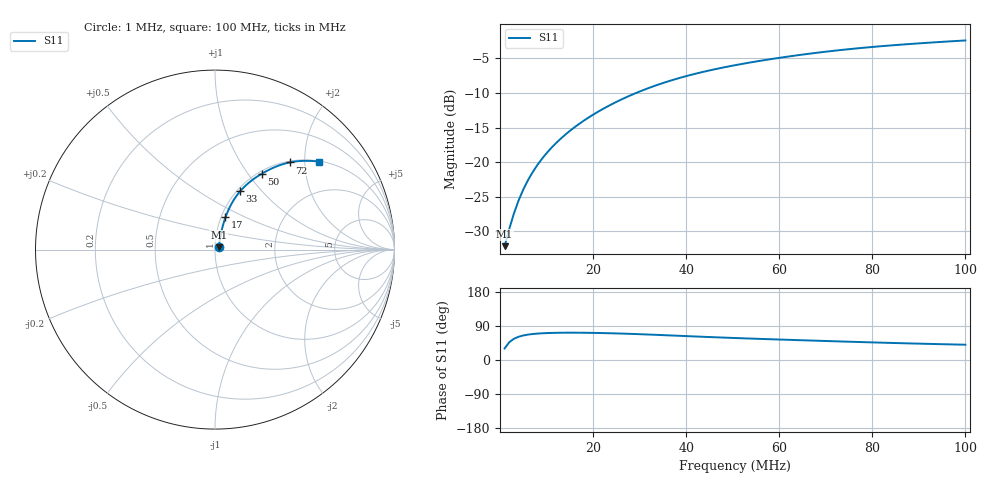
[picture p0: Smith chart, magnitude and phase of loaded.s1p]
# MHz S RI R 50.0
! SimSmith 18.4f
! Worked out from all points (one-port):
!   100 points, 1 MHz to 100 MHz, reference 50 ohm
!   lowest |S11| = -32.1 dB at 1 MHz (marker M1), VSWR 1.05, Z = 52.2 + j1.31 ohm
!   |S11| at or under -10 dB: start of sweep to 29.24 MHz
!   S11 on the Smith chart (normalised r, x): 1 MHz: 1.04, +0.03; 17 MHz: 1.05, +0.39; 33 MHz: 1.04, +0.77; 50 MHz: 1.04, +1.17; 72 MHz: 1.02, +1.69; 100 MHz: 1.02, +2.34
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1  0.0213 0.0125
2  0.0225 0.0241
3  0.0239 0.0353
4  0.0254 0.0464
5  0.027 0.0573
6  0.0289 0.068
7  0.0309 0.0786
8  0.033 0.0891
9  0.0353 0.0994
11  0.0403 0.1199
12  0.0429 0.13
14  0.0487 0.15
17  0.0585 0.1797
21  0.0739 0.2186
23  0.0828 0.2376
26  0.0978 0.2655
29  0.1148 0.2921
33  0.1401 0.3249
39  0.1822 0.3671
44  0.2188 0.3958
50  0.2624 0.4239
51  0.2695 0.428
57  0.3121 0.45
63  0.3542 0.4678
72  0.4166 0.4858
76  0.4432 0.4903
88  0.5158 0.4944
100  0.578 0.4906
